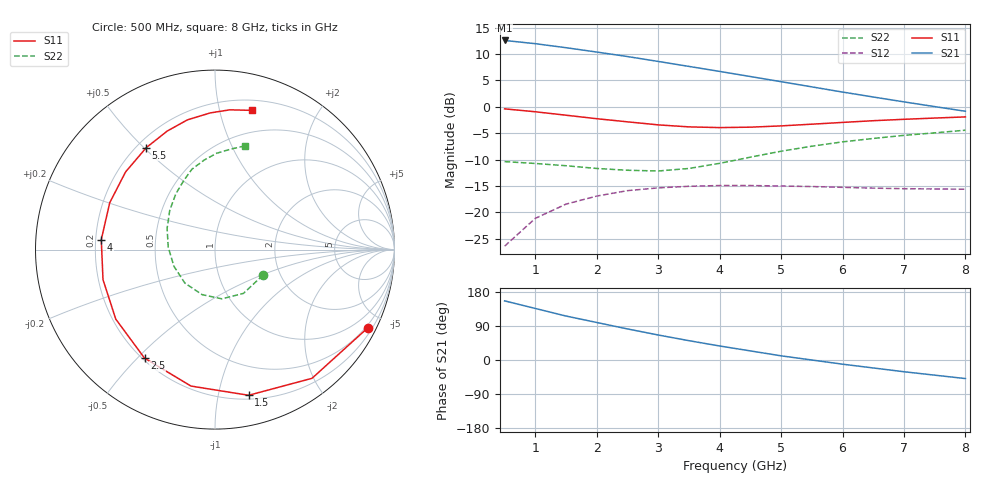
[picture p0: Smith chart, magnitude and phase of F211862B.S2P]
!ATF-21186
!S-PARAMETERS at Vds=2V  Id=15mA.  LAST UPDATED 01-30-98
# ghz s ma r 50
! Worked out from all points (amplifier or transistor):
!   16 points, 500 MHz to 8 GHz, reference 50 ohm
!   highest |S21| = 12.6 dB at 500 MHz (marker M1)
!   |S21| within 3 dB of that: start of sweep to 2.474 GHz
!   unconditionally stable (mu >= 1): 5.853 GHz to end of sweep
!   at 1.5 GHz: K = 0.37, MSG = 14.8 dB, |S12| = -18.4 dB
!   at 4.5 GHz: K = 0.88, MSG = 10.3 dB, |S12| = -14.9 dB
!   at 8 GHz: K = 1.05, MAG = 6.0 dB, |S12| = -15.6 dB
!   lowest NFmin = 0.35 dB at 500 MHz
!   S11 on the Smith chart (normalised r, x): 500 MHz: 0.40, -4.13; 1.5 GHz: 0.23, -1.23; 2.5 GHz: 0.21, -0.52; 4 GHz: 0.22, +0.04; 5.5 GHz: 0.24, +0.51; 8 GHz: 0.29, +1.26
0.5  0.957 -27.0  4.248 156.0  0.048 71.0  0.303 -28.0
1  0.898 -53.0  3.959 136.0  0.088 57.0  0.291 -57.0
1.5  0.833 -77.0  3.627 116.0  0.12 44.0  0.277 -82.0
2  0.772 -100.0  3.3 99.0  0.143 32.0  0.261 -106.0
2.5  0.721 -123.0  2.992 82.0  0.161 22.0  0.251 -132.0
3  0.675 -145.0  2.689 66.0  0.171 12.0  0.247 -158.0
3.5  0.646 -165.0  2.413 51.0  0.177 3.0  0.261 177.0
4  0.636 175.0  2.164 37.0  0.18 -4.0  0.292 156.0
4.5  0.642 156.0  1.936 24.0  0.18 -11.0  0.334 139.0
5  0.66 139.0  1.73 11.0  0.178 -17.0  0.38 125.0
5.5  0.685 124.0  1.545 0.0  0.176 -23.0  0.424 114.0
6  0.712 112.0  1.38 -11.0  0.173 -27.0  0.466 106.0
6.5  0.739 102.0  1.239 -21.0  0.17 -32.0  0.502 97.0
7  0.762 92.0  1.114 -31.0  0.168 -36.0  0.537 89.0
7.5  0.783 84.0  1.005 -40.0  0.167 -39.0  0.567 81.0
8  0.803 75.0  0.908 -49.0  0.166 -44.0  0.601 74.0
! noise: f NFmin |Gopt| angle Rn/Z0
0.5  0.35  0.95  13  1.633
1  0.39  0.87  27  0.639
2  0.46  0.76  63  0.302
3  0.54  0.67  102  0.138
3.5  0.57  0.635  121  0.088
4.5  0.64  0.605  165  0.025
5.5  0.72  0.65  -152  0.042
6  0.75  0.696  -136  0.088
7  0.83  0.782  -109  0.301
8  0.9  0.84  -86  0.715
